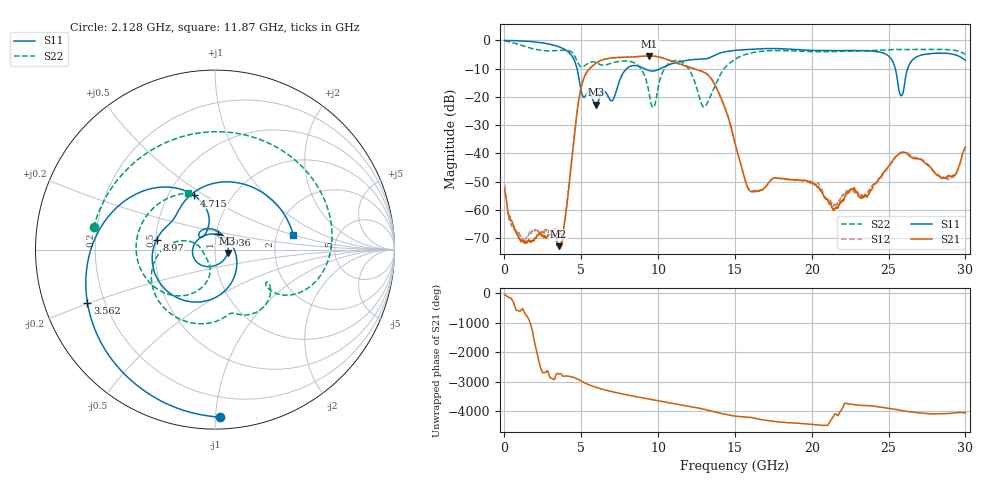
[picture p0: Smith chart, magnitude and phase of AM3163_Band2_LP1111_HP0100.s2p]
!Agilent Technologies,E8364B,MY43040894,A.07.50.67
!Agilent E8364B: A.07.50.67
!Date: Thursday, August 20, 2020 12:07:33
!Correction: S11(Full 2 Port(1,2))
!S21(Full 2 Port(1,2))
!S12(Full 2 Port(1,2))
!S22(Full 2 Port(1,2))
!S2P File: Measurements: S11, S21, S12, S22:
# Hz S  dB  R 50
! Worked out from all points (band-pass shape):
!   3201 points, 10 MHz to 30 GHz, reference 50 ohm
!   highest |S21| = -5.48 dB at 9.429 GHz (marker M1); lowest = -72.9 dB at 3.524 GHz (marker M2)
!   |S21| within 3 dB of the highest: 5.849 GHz to 11.5 GHz (5.654 GHz wide, 65.2 % of centre)
!   lowest |S11| = -22.8 dB at 5.942 GHz (marker M3), VSWR 1.16, Z = 57.5 - j2.19 ohm
!   |S11| at or under -10 dB: 4.723 GHz to 7.957 GHz (3.234 GHz wide, 51 % of centre); 9.115 GHz to 10.14 GHz (1.027 GHz wide, 10.7 % of centre); 25.44 GHz to 26.24 GHz (801.6 MHz wide, 3.1 % of centre)
!   |S22| runs from -23.8 to -0.1 dB; largest |S21 - S12| = 0.013
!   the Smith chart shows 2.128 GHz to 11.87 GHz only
!   S11 on the Smith chart (normalised r, x): 2.128 GHz: 0.07, -1.03; 3.562 GHz: 0.14, -0.20; 4.715 GHz: 0.67, +0.45; 6.936 GHz: 1.01, +0.17; 8.97 GHz: 0.51, +0.06; 11.87 GHz: 2.48, +0.50
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1e7  0.01 -2.7  -52.71 -50.5  -51.10 109.6  -0.14 -6.7
9.190719e8  -0.10 -37.3  -69.82 115.3  -67.55 113.2  -1.40 -88.5
2.128044e9  -0.59 -88.2  -69.15 125.2  -66.92 32.6  -3.25 169.6
3.524453e9  -2.20 -155.3  -72.91 153.6  -67.33 -139.7  -3.55 61.9
3.561941e9  -2.27 -157.4  -72.62 151.7  -68.55 96.0  -3.54 59.0
4.714681e9  -9.81 111.1  -25.79 -16.5  -25.81 -16.9  -7.16 -34.7
5.014581e9  -18.42 110.2  -16.07 -101.3  -16.09 -101.6  -9.40 -33.4
5.942397e9  -22.79 -15.2  -8.10 55.1  -8.14 54.9  -7.82 -63.1
6.935816e9  -21.36 80.5  -6.24 -87.8  -6.29 -88.0  -8.08 -86.8
8.969512e9  -9.62 170.3  -5.60 58.9  -5.58 58.9  -10.81 179.2
9.428734e9  -10.71 150.3  -5.48 13.9  -5.46 13.7  -19.10 163.5
1.000979e10  -10.34 129.6  -5.80 -43.6  -5.84 -44.2  -16.35 -102.3
1.186542e10  -7.05 10.5  -9.15 143.8  -9.19 145.6  -9.16 115.7
1.300879e10  -6.57 -50.1  -11.33 27.8  -11.28 29.3  -23.57 -103.4
1.5005e10  -3.51 -132.8  -36.41 159.3  -36.40 159.2  -6.70 -112.1
1.598905e10  -3.17 -173.7  -53.30 116.8  -52.90 117.4  -4.53 -171.5
1.787279e10  -2.89 98.1  -48.88 -38.5  -48.86 -38.2  -3.58 92.2
2.000958e10  -3.51 -9.8  -50.30 -122.1  -50.99 -120.1  -3.94 -9.4
2.231506e10  -3.55 -100.1  -54.15 -143.3  -53.26 -138.4  -3.86 -93.7
2.500479e10  -5.54 157.7  -44.51 66.4  -44.86 69.7  -3.35 -167.5
2.582014e10  -19.55 170.5  -39.73 -8.7  -39.66 -6.6  -3.21 170.4
3e10  -6.98 50.9  -37.80 -85.3  -37.94 -85.6  -4.80 55.6
